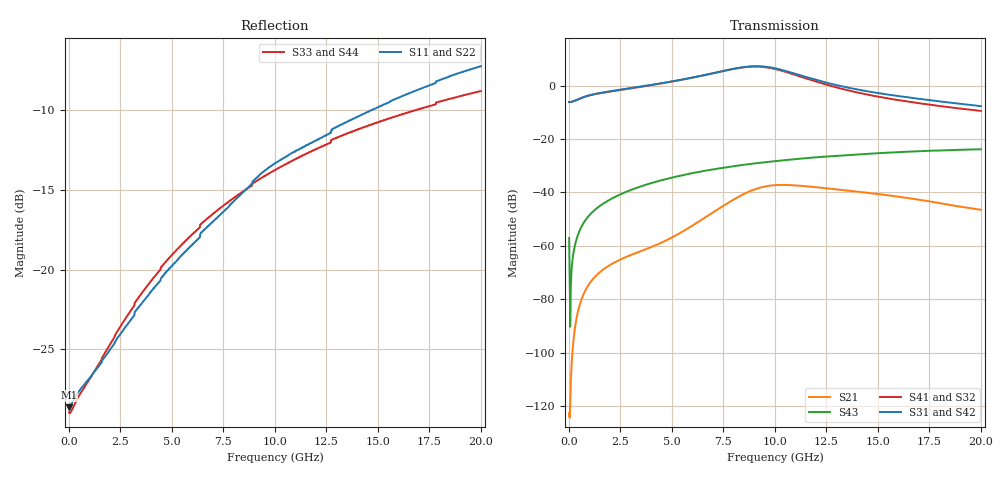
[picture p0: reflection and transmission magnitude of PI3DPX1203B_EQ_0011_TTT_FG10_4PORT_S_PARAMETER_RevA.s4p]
! NPort=4 DATA=2000 NOISE=0 GROUPDELAY=0 COMPLEX_DATAFORMAT=POLAR
! NumOfBlock=1 NumOfParam=0
! .MODEL Smodel S TSTONEFILE=PI3DPX1203B_EQ_0011_TTT_FG10_4PORT_S_PARAMETER_RevA.s4p TYPE=S
!  -- The above .MODEL line can be used for the S element in the netlist.
! The s parameter is extracted from the linear redriver, it is not bi-directional; only s(4,1)s(4,2) and s(3,1)s(3,2)
! should be the insertion loss
!Port definition:
!Port1 = input+
!Port2 = input-
!Port3 = output+
!Port4 = output-
# Hz S MA R  50
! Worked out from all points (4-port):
!   2000 points, 10 MHz to 20 GHz, reference 50 ohm
!   strongest paths, dB at 10 MHz, 5.01 GHz, 10.01 GHz, 15.01 GHz, 20 GHz:
!     S31: -6.2, 1.6, 6.5, -2.8, -7.7
!     S42: -6.2, 1.6, 6.5, -2.8, -7.7
!     S41: -6.2, 1.5, 6.2, -4.1, -9.5
!     S32: -6.2, 1.5, 6.2, -4.1, -9.5
!     S43: -57.1, -34.4, -28.3, -25.3, -23.8
!     S21: -122.7, -56.8, -37.3, -40.6, -46.5
!   lowest |S11| = -28.6 dB at 10 MHz (marker M1), VSWR 1.08, Z = 46.4 - j0.0306 ohm
!   |S11| at or under -10 dB: start of sweep to 14.67 GHz
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1e7  0.03701 -179.5  7.338e-07 10.6  0 0.0  0 0.0
     7.338e-07 10.6  0.03701 -179.5  0 0.0  0 0.0
     0.4917 -0.1  0.4917 179.9  0.03566 178.2  0.001403 -77.8
     0.4917 179.9  0.4917 -0.1  0.001403 -77.8  0.03566 178.2
1.58e9  0.05108 -144.6  0.0003395 114.3  5.314e-12 74.8  5.089e-11 115.5
        0.0003395 114.3  0.05108 -144.6  5.089e-11 115.5  5.314e-12 74.8
        0.7354 3.1  0.7286 -177.0  0.05212 -142.0  0.005859 82.8
        0.7286 -177.0  0.7354 3.1  0.005859 82.8  0.05212 -142.0
6.18e9  0.1233 -111.0  0.002653 135.5  1.741e-08 -113.9  1.576e-07 66.0
        0.002652 135.5  0.1233 -111.0  1.575e-07 66.0  1.741e-08 -113.9
        1.462 -47.8  1.457 134.5  0.1325 -116.9  0.02371 64.3
        1.458 134.5  1.461 -47.8  0.02371 64.3  0.1325 -116.9
8.6e9  0.1789 -106.0  0.009779 105.1  4.17e-07 158.6  1.161e-06 16.5
       0.009774 105.2  0.1789 -106.0  1.159e-06 16.5  4.17e-07 158.6
       2.252 -101.5  2.224 80.4  0.1787 -115.9  0.03336 51.8
       2.225 80.4  2.251 -101.5  0.03336 51.8  0.1787 -115.9
1.006e10  0.2168 -107.3  0.01374 62.6  1.311e-06 96.2  2.268e-06 -21.4
          0.01373 62.6  0.2168 -107.3  2.265e-06 -21.3  1.312e-06 96.2
          2.089 -149.0  2.02 32.7  0.2065 -116.3  0.0387 44.0
          2.022 32.7  2.087 -148.9  0.0387 44.0  0.2065 -116.3
1.219e10  0.2588 -108.7  0.0123 19.7  3.146e-06 30.6  4.063e-06 -49.3
          0.01229 19.8  0.2588 -108.7  4.063e-06 -49.1  3.147e-06 30.6
          1.225 166.4  1.128 -11.2  0.2421 -117.6  0.04606 33.2
          1.13 -11.2  1.224 166.5  0.04606 33.2  0.2421 -117.6
2e10  0.4355 -116.6  0.004708 -23.6  2.197e-05 -106.5  3.241e-05 -134.0
      0.004734 -23.4  0.4355 -116.6  3.249e-05 -133.9  2.2e-05 -106.4
      0.4126 83.9  0.3362 -78.3  0.3637 -123.9  0.06431 -7.1
      0.3357 -78.5  0.4132 83.9  0.06431 -7.1  0.3637 -123.9
